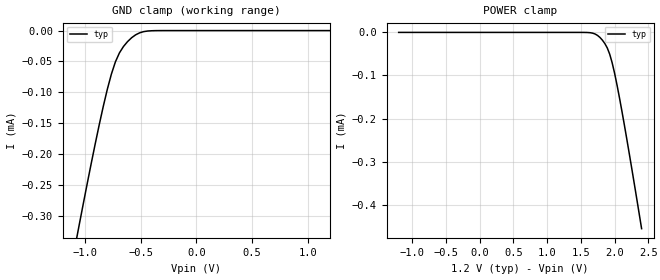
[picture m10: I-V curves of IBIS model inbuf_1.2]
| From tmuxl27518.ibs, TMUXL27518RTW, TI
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| inbuf_1.2
[Model]   inbuf_1.2
Model_type   Input
Vinl = 0.39
Vinh = 0.77
|   typ   min   max
C_comp   2.533030e-13   NA   NA
[Voltage Range]   1.2   NA   NA
[Temperature Range]   27   NA   NA
[Power Clamp Reference]   1.2   NA   NA
[GND Clamp Reference]   0   NA   NA
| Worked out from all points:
|   GND clamp passes 1 mA (typ) near -1.75 V on its own axis
[GND Clamp]
|   Voltage   I(typ)   I(min)   I(max)
-2.4V     -1.666mA   NA         NA
-1.091V   -350.8uA   NA         NA
-1.055V   -316.4uA   NA         NA
-872.7mV  -152.5uA   NA         NA
-800mV    -95.05uA   NA         NA
-763.6mV  -70.55uA   NA         NA
-727.3mV  -50.58uA   NA         NA
-690.9mV  -35.99uA   NA         NA
-618.2mV  -17.84uA   NA         NA
-545.5mV  -6.858uA   NA         NA
-363.6mV  -86.02nA   NA         NA
1.2V      83.05pA    NA         NA
[POWER Clamp]
|   Voltage   I(typ)   I(min)   I(max)
-1.2V     16.5nA     NA         NA
1.564V    -86.02nA   NA         NA
1.673V    -1.66uA    NA         NA
1.745V    -6.858uA   NA         NA
1.818V    -17.84uA   NA         NA
1.891V    -35.99uA   NA         NA
1.927V    -50.58uA   NA         NA
2V        -95.05uA   NA         NA
2.073V    -152.5uA   NA         NA
2.145V    -215.8uA   NA         NA
2.255V    -316.4uA   NA         NA
2.4V      -455.8uA   NA         NA
